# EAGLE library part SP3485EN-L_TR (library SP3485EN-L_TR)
RS-485 Interface IC 3.3V LoPwr Half-Dup RS485w/10Mbps Data Source: Datasheet
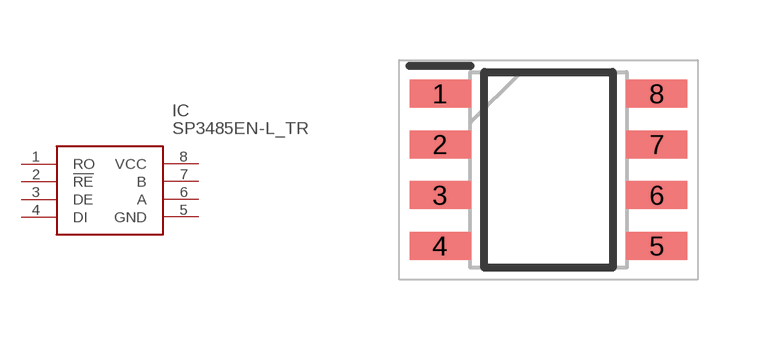
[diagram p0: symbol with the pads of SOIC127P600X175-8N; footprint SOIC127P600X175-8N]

Designator prefix IC

## SP3485EN-L_TR (Description: RS-485 Interface IC 3.3V LoPwr Half-Dup RS485w/10Mbps Data; Height: 1.75mm; Manufacturer_Name: MaxLinear, Inc.; Manufacturer_Part_Number: SP3485EN-L/TR; Mouser_Part_Number: 701-SP3485EN-L/TR; Mouser_Price-Stock: https://www.mouser.co.uk/ProductDetail/MaxLinear/SP3485EN-L-TR?qs=3EMgrMjM0fbQ17liGrle%2Fg%3D%3D)  [SOIC127P600X175-8N]
1  RO
2  !RE
3  DE
4  DI
5  GND
6  A
7  B
8  VCC

## Footprint SOIC127P600X175-8N (pad centres in mm)
SP2525A-1EN-L/TR-1
smd 1.525 x 0.7: 1 -2.712,1.905; 2 -2.712,0.635; 3 -2.712,-0.635; 4 -2.712,-1.905; 5 2.712,-1.905; 6 2.712,-0.635; 7 2.712,0.635; 8 2.712,1.905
